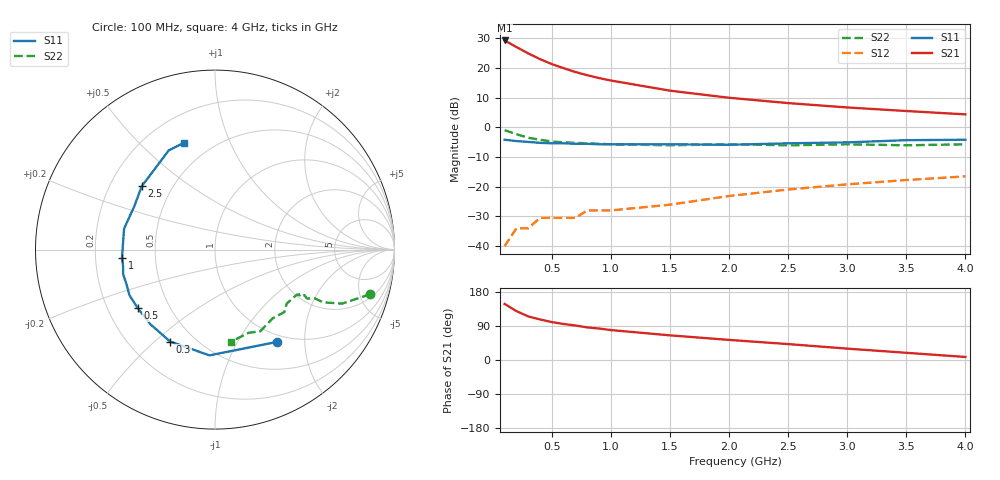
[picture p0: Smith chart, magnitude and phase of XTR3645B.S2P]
! HXTR-3645 Common Emitter
! Vce=15V  Ic=18mA
# ghz s ma r 50
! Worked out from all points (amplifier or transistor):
!   16 points, 100 MHz to 4 GHz, reference 50 ohm
!   highest |S21| = 29.3 dB at 100 MHz (marker M1)
!   |S21| within 3 dB of that: start of sweep to 236.6 MHz
!   unconditionally stable (mu >= 1): 1.128 GHz to 2.53 GHz
!   at 300 MHz: K = 0.47, MSG = 29.5 dB, |S12| = -34.0 dB
!   at 900 MHz: K = 0.85, MSG = 22.3 dB, |S12| = -28.0 dB
!   at 4 GHz: K = 0.77, MSG = 10.4 dB, |S12| = -16.5 dB
!   S11 on the Smith chart (normalised r, x): 100 MHz: 0.89, -1.49; 300 MHz: 0.37, -0.56; 500 MHz: 0.33, -0.30; 1 GHz: 0.32, -0.04; 2.5 GHz: 0.34, +0.34; 4 GHz: 0.36, +0.69
0.1  0.62 -56.0  29.17 148.0  0.01 69.0  0.9 -16.0
0.2  0.59 -93.0  22.6 129.0  0.02 66.0  0.77 -23.0
0.3  0.57 -116.0  17.66 115.0  0.02 50.0  0.67 -26.0
0.4  0.55 -131.0  14.14 107.0  0.03 55.0  0.62 -26.0
0.5  0.54 -143.0  11.65 100.0  0.03 47.0  0.58 -28.0
0.6  0.54 -152.0  9.96 95.0  0.03 48.0  0.56 -27.0
0.7  0.53 -158.0  8.57 91.0  0.03 51.0  0.55 -28.0
0.8  0.53 -165.0  7.57 86.0  0.04 52.0  0.54 -29.0
0.9  0.52 -170.0  6.78 83.0  0.04 57.0  0.53 -28.0
1  0.52 -175.0  6.16 79.0  0.04 57.0  0.52 -29.0
1.5  0.52 167.0  4.16 65.0  0.05 59.0  0.5 -37.0
2  0.51 152.0  3.16 53.0  0.07 63.0  0.52 -42.0
2.5  0.54 139.0  2.57 42.0  0.09 64.0  0.5 -50.0
3  0.56 127.0  2.17 30.0  0.11 62.0  0.52 -61.0
3.5  0.61 115.0  1.89 19.0  0.13 59.0  0.5 -68.0
4  0.62 106.0  1.66 8.0  0.15 55.0  0.52 -80.0
